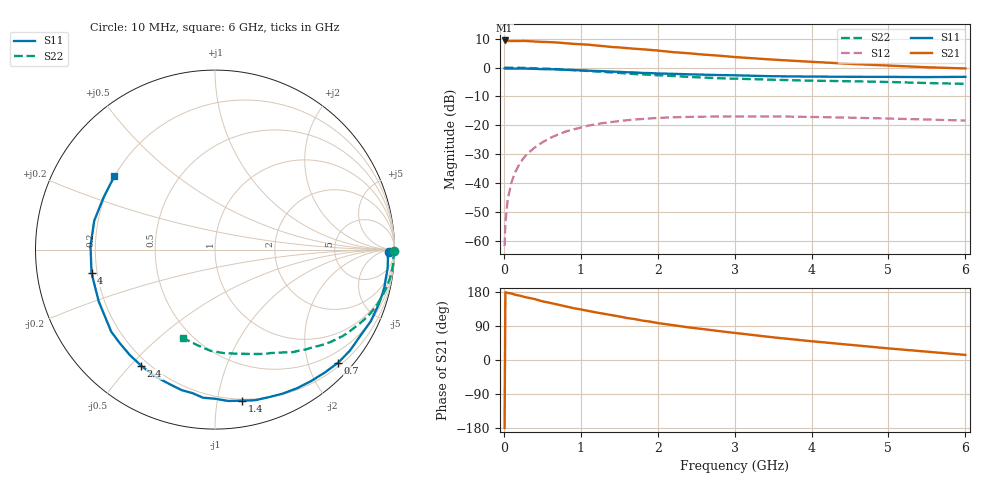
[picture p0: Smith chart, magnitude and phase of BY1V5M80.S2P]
! SIEMENS Small Signal Semiconductors
! BFY420
! Si NPN RF SIEGET Grounded Emitter Transistor in MICRO-X
! VCE = 1.5 V  IC = 0.8 mA
! Common Emitter S-Parameters:  October  1996
# GHz  S  MA  R  50
!  f  S11  S21  S12  S22
! GHz  MAG  ANG  MAG  ANG  MAG  ANG  MAG  ANG
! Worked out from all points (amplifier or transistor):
!   36 points, 10 MHz to 6 GHz, reference 50 ohm
!   highest |S21| = 9.4 dB at 10 MHz (marker M1)
!   |S21| within 3 dB of that: start of sweep to 1.767 GHz
!   unconditionally stable (mu >= 1): 4.661 GHz to end of sweep
!   at 250 MHz: K = 0.04, MSG = 20.4 dB, |S12| = -31.6 dB
!   at 1.4 GHz: K = 0.20, MSG = 13.0 dB, |S12| = -18.9 dB
!   at 6 GHz: K = 1.36, MAG = 5.5 dB, |S12| = -18.4 dB
!   S11 on the Smith chart (normalised r, x): 10 MHz: 54, -24; 700 MHz: 0.27, -2.55; 1.4 GHz: 0.19, -1.18; 2.4 GHz: 0.17, -0.54; 4 GHz: 0.18, -0.09; 6 GHz: 0.20, +0.31
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0.01  0.9697 -0.8  2.964 -179.2  0.0008 99.2  0.9992 -0.3
0.02  0.9615 -1.3  2.945 178.7  0.002 95.5  0.9995 -0.6
0.05  0.9649 -3.1  2.9 177.1  0.0052 91.9  0.9978 -1.6
0.1  0.9675 -6.3  2.907 175.5  0.0103 87.0  0.9939 -3.2
0.15  0.9651 -9.3  2.894 171.9  0.0156 83.5  0.9953 -4.8
0.2  0.967 -12.5  2.896 170.2  0.0208 83.1  0.9935 -6.2
0.3  0.962 -18.4  2.897 164.9  0.0315 79.3  0.9876 -9.4
0.4  0.9552 -24.7  2.842 160.8  0.0411 74.6  0.9782 -12.5
0.5  0.9414 -30.8  2.8 154.9  0.0506 70.7  0.9678 -15.5
0.7  0.9317 -42.5  2.726 146.3  0.0688 63.8  0.9414 -21.3
0.9  0.9072 -53.9  2.589 137.1  0.0846 56.2  0.9085 -26.6
1.1  0.8864 -65.0  2.502 129.5  0.0989 49.7  0.8753 -31.7
1.4  0.8547 -79.9  2.283 118.4  0.1139 40.8  0.8265 -38.4
1.8  0.8093 -99.0  2.083 104.0  0.1285 30.5  0.7638 -45.8
2.2  0.7819 -115.2  1.859 91.9  0.1377 21.7  0.7179 -52.7
2.4  0.7667 -122.4  1.778 86.1  0.1397 18.3  0.6913 -55.9
2.8  0.7434 -135.7  1.614 76.2  0.1424 11.7  0.6556 -61.5
3.5  0.7093 -156.0  1.378 59.8  0.1428 2.8  0.6171 -70.5
4  0.7 -169.3  1.263 49.5  0.1396 -2.0  0.5941 -77.4
4.5  0.6939 178.4  1.164 40.1  0.1357 -6.1  0.5806 -84.4
5.5  0.6855 154.7  1.016 22.0  0.1259 -10.4  0.5409 -100.7
6  0.6938 143.9  0.968 13.4  0.1209 -10.6  0.5235 -110.0
